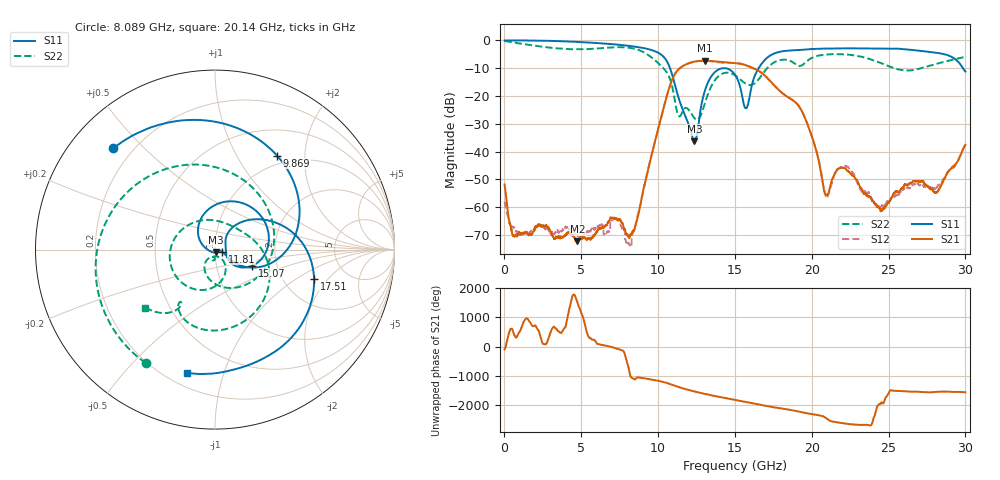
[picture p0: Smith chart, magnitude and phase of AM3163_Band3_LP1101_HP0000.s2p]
!Agilent Technologies,E8364B,MY43040894,A.07.50.67
!Agilent E8364B: A.07.50.67
!Date: Thursday, August 20, 2020 12:11:45
!Correction: S11(Full 2 Port(1,2))
!S21(Full 2 Port(1,2))
!S12(Full 2 Port(1,2))
!S22(Full 2 Port(1,2))
!S2P File: Measurements: S11, S21, S12, S22:
# Hz S  dB  R 50
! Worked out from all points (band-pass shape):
!   3201 points, 10 MHz to 30 GHz, reference 50 ohm
!   highest |S21| = -7.27 dB at 13.04 GHz (marker M1); lowest = -72.3 dB at 4.752 GHz (marker M2)
!   |S21| within 3 dB of the highest: 11.35 GHz to 16.3 GHz (4.951 GHz wide, 35.8 % of centre)
!   lowest |S11| = -36.2 dB at 12.36 GHz (marker M3), VSWR 1.03, Z = 50.5 - j1.47 ohm
!   |S11| at or under -10 dB: 10.78 GHz to 14.2 GHz (3.422 GHz wide, 27.4 % of centre); 14.39 GHz to 16.54 GHz (2.155 GHz wide, 13.9 % of centre); 29.84 GHz to end of sweep
!   |S22| runs from -28.6 to -0.2 dB; largest |S21 - S12| = 0.014
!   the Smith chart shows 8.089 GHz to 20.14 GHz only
!   S11 on the Smith chart (normalised r, x): 8.089 GHz: 0.13, +0.41; 9.869 GHz: 0.86, +1.49; 11.81 GHz: 1.08, -0.02; 15.07 GHz: 1.49, -0.28; 17.51 GHz: 2.95, -1.43; 20.14 GHz: 0.28, -0.76
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1e7  -0.02 -2.2  -51.87 -95.1  -58.00 -41.7  -0.19 -5.5
1.172112e9  -0.00 -32.1  -69.68 23.9  -69.27 -5.0  -1.25 -82.4
2.512291e9  -0.09 -68.9  -66.71 96.9  -67.03 -71.2  -2.30 -161.5
4.752169e9  -0.54 -128.6  -72.32 65.8  -70.33 123.0  -3.20 79.6
5.014581e9  -0.61 -135.6  -71.02 37.1  -70.35 151.6  -3.19 65.4
6.504709e9  -1.12 -176.3  -66.94 40.4  -69.81 1.4  -2.70 -19.6
8.088556e9  -1.94 135.0  -70.94 -28.0  -73.21 24.5  -2.61 -121.4
9.869212e9  -4.05 56.5  -34.80 -76.5  -34.83 -77.0  -7.48 69.9
1.000979e10  -4.43 47.6  -31.75 -91.5  -31.82 -91.9  -8.19 49.8
1.180919e10  -27.74 -16.3  -8.62 -20.1  -8.65 -19.9  -24.26 -100.6
1.236213e10  -36.25 -70.4  -7.62 -96.9  -7.64 -96.8  -27.94 -102.9
1.303691e10  -18.21 139.2  -7.27 179.8  -7.30 179.3  -22.75 -53.8
1.5005e10  -12.34 -19.0  -8.15 -24.1  -8.12 -22.2  -12.56 166.7
1.50706e10  -12.92 -23.4  -8.19 -30.7  -8.13 -28.9  -12.82 160.6
1.573601e10  -24.39 9.8  -8.98 -98.6  -8.88 -98.3  -15.65 94.8
1.750729e10  -4.80 -16.4  -15.87 83.9  -15.91 84.9  -8.04 -48.8
2.000958e10  -3.09 -99.4  -34.63 -150.8  -34.59 -150.6  -6.25 -135.3
2.014079e10  -3.06 -102.8  -36.83 -161.8  -36.80 -161.9  -5.93 -140.2
2.094677e10  -2.92 -122.4  -55.62 63.6  -56.11 -150.1  -5.06 -169.7
2.217448e10  -2.85 -150.2  -46.05 -113.7  -45.16 -112.5  -4.99 146.7
2.500479e10  -2.99 144.2  -58.33 -160.1  -58.01 -50.7  -9.27 13.5
3e10  -11.17 -30.4  -37.58 -123.1  -37.89 -123.9  -5.95 119.3
